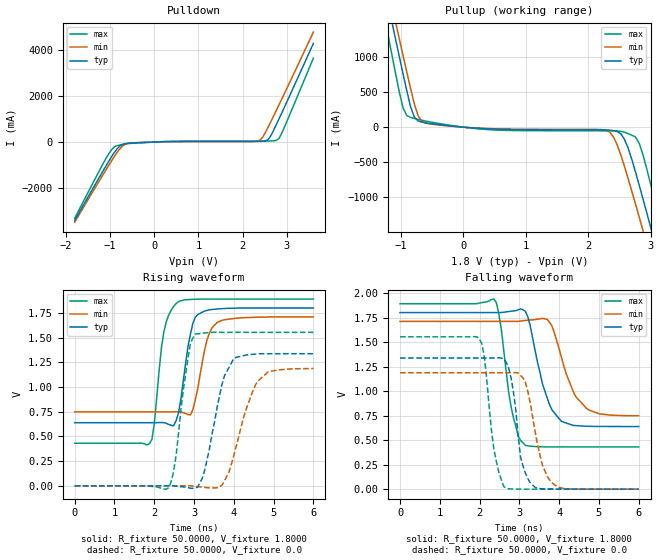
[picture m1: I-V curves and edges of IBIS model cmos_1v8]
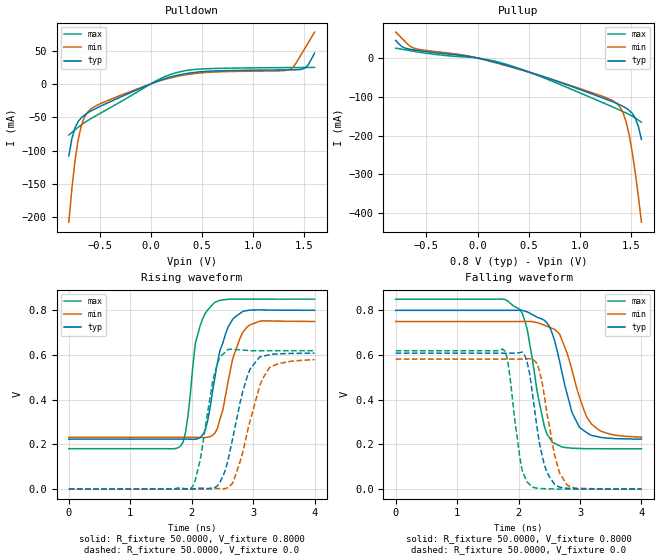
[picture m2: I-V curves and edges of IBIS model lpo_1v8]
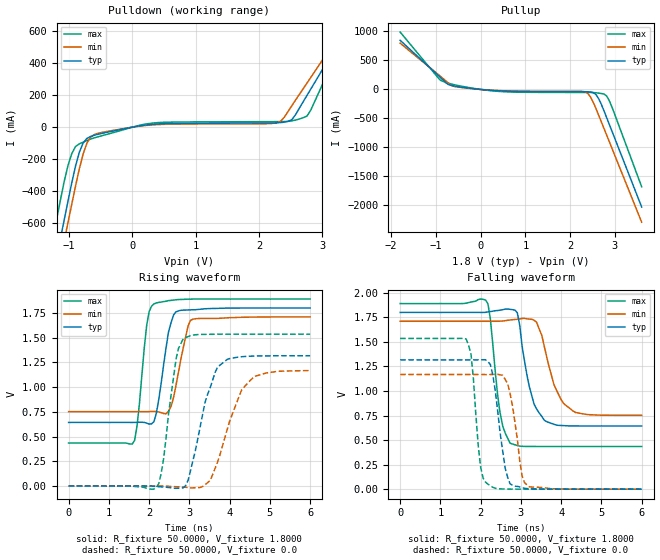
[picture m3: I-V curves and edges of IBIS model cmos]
[IBIS ver]   4.1
[File name]   5l35023.ibs
[File Rev]   1.1
[Date]   Mar 30, 2017
[Source]   IDT
[Notes]   1. Temp typ=25C, max=105C, min=-40C
[Disclaimer]
READ THESE TERMS AND CONDITIONS CAREFULLY BEFORE USING THIS IBIS MODEL.  BY
USING THIS IBIS MODEL, YOU ARE ACCEPTING AND AGREEING TO THESE TERMS AND
CONDITIONS OF USE.
INTEGRATED DEVICE TECHNOLOGY, INC. ("IDT") HEREBY GRANTS THE USER OF THIS
IBIS MODEL ("USER") A NON-EXCLUSIVE, NONTRANSFERABLE LICENSE TO USE THIS
IBIS MODEL UNDER THE FOLLOWING TERMS: THE USER IS GRANTED THIS LICENSE ONLY
TO USE THE IBIS MODEL FOR DEMONSTRATION PURPOSES ONLY AND IS NOT GRANTED
RIGHTS TO SELL, COPY (EXCEPT AS NEEDED TO RUN THE IBIS MODEL), RENT, LEASE
OR SUB-LICENSE (EXCEPT FOR DEMONSTRATION) THE IBIS MODEL IN WHOLE OR IN
PART, OR IN MODIFIED FORM TO ANYONE. THE USER MAY MODIFY THE IBIS MODEL TO
SUIT ITS SPECIFIC APPLICATIONS, BUT  RIGHTS TO DERIVATIVE WORKS AND SUCH
MODIFICATIONS SHALL BELONG TO IDT.
THIS IBIS MODEL IS PROVIDED ON AN AS IS" BASIS AND IDT  MAKES ABSOLUTELY NO
WARRANTY WITH RESPECT TO THE INFORMATION CONTAINED HEREIN.  IDT DISCLAIMS
AND USER WAIVES ALL WARRANTIES, EXPRESS AND IMPLIED, INCLUDING WARRANTIES OF
MERCHANTABILITY AND FITNESS FOR A PARTICULAR PURPOSE.  THE ENTIRE RISK AS TO
QUALITY AND PERFORMANCE IS WITH THE USER  ACCORDINGLY, IN NO EVENT SHALL IDT
BE LIABLE FOR ANY DIRECT OR INDIRECT DAMAGES, WHETHER IN CONTRACT OR TORT,
INCLUDING ANY LOST PROFITS OR OTHER INCIDENTAL, CONSEQUENTIAL, EXEMPLARY, OR
PUNITIVE DAMAGES ARISING OUT OF THE USE OR APPLICATION OF THE  IBIS MODEL,
WHETHER OR NOT IDT HAD NOTICE OF SUCH DAMAGES.
IDT RESERVES THE RIGHT TO MAKE CHANGES WITHOUT NOTICE TO ANY PRODUCT HEREIN
TO IMPROVE RELIABILITY, FUNCTION, OR DESIGN. IDT DOES NOT CONVEY ANY LICENSE
UNDER PATENT RIGHTS OR ANY OTHER INTELLECTUAL PROPERTY RIGHTS, INCLUDING
THOSE OF THIRD PARTIES. IDT IS NOT OBLIGATED TO PROVIDE  MAINTENANCE OR
SUPPORT FOR THE LICENSED IBIS MODEL.
This model is for VC3S 1.8V in 24 pin package
[Copyright]
Copyright 2017, Integrated Device Technology, Inc. All rights  reserved.
|History
|Rev 1.0 Created on Feb 22, 2017
|Rev 1.1 Fixed pinout, Mar 30, 2017
|   Component IDT_vc3s_1p8v
[Component]   IDT_vc3s_1p8v
[Manufacturer]   Integrated Device Technology Inc.
[Package]
| Following package parameters are for the 24 pin QFN package
| variable   typ   min   max
R_pkg   72.4655m   58.886m   86.045m
L_pkg   1.47175nH   1.11650nH   1.77850nH
C_pkg   0.07747pF   0.07444pF   0.08050pF
[Pin]  signal_name   model_name
1   VDDA   POWER
2   SDA   input
3   SCL   input
4   X2   NC
5   XIN   xin
6   VBAT   POWER
7   NC   NC
8   REF   cmos
9   VDD18   POWER
10   OE2   input
11   VDDSE2   POWER
12   SE2   cmos
13   VDDSE1   POWER
14   SE1   cmos
15   OE1   input
16   VDDDIFF1   POWER
17   DIFF1B   IO
18   DIFF1   IO
19   SE3   cmos
20   VDDSE3   POWER
21   OE3   input
22   VDDDIFF2   POWER
23   DIFF2B   IO
24   DIFF2   IO
25   EPAD   GND
[Diff Pin]  inv_pin  vdiff   tdelay_typ  tdelay_min  tdelay_max
18   17   0.000V   0.000s   0.000s   0.000s
24   23   0.000V   0.000s   0.000s   0.000s
[Model Selector] IO
cmos_1v8  1.8V LVCMOS
lpo_1v8   1.8V LP-HCSL
| Models and submodels in the file (5): cmos_1v8 (Output), lpo_1v8 (Output), cmos (Output), input (Input), xin (Input)
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|   Model CMOS_1V8
[Model]  cmos_1v8
Model_type Output
Polarity   Non-Inverting
Vmeas =  0.9000V
Cref =   5.0000pF
Rref =   50.0000
Vref =   0.9000V
C_comp   2.0000pF   1.5000pF   2.5000pF
[Temperature Range]   55.0000   0.1050k   -40.0000
[Voltage Range]   1.8000V   1.7100V   1.8900V
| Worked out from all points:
|   slope of the pulldown table from 0 to 0.27 V, typ, clamps not added: 17.2 ohm
|   slope of the pullup table from 0 to 0.27 V, typ, clamps not added: 15 ohm
|   rising waveform, R_fixture 50.0000, V_fixture 1.8000: 20-80 % time 261ps typ, 293ps min, 242ps max; typ from 0.639 V to 1.8 V
|   rising waveform, R_fixture 50.0000, V_fixture 0.0: 20-80 % time 405ps typ, 518ps min, 280ps max; typ from 0 V to 1.34 V
|   falling waveform, R_fixture 50.0000, V_fixture 1.8000: 20-80 % time 429ps typ, 489ps min, 299ps max; typ from 1.8 V to 0.639 V
|   falling waveform, R_fixture 50.0000, V_fixture 0.0: 20-80 % time 252ps typ, 350ps min, 260ps max; typ from 1.34 V to 0 V
[Pulldown]
|Voltage   I(typ)   I(min)   I(max)
-1.8V     -3.421A    -3.497A    -3.324A
-1.02V    -808.5mA   -987.3mA   -484.5mA
-900mV    -444.5mA   -622.2mA   -206mA
-720mV    -106.4mA   -182.2mA   -104.7mA
-480mV    -39.39mA   -33.93mA   -53.82mA
2.22V     26.08mA    23.46mA    34.43mA
2.4V      30.69mA    93.67mA    34.93mA
2.58V     118.4mA    663.2mA    42.95mA
2.76V     754.3mA    1.372A     69.48mA
2.82V     1A         1.613A     152.6mA
3V        1.752A     2.341A     897.6mA
3.6V      4.301A     4.795A     3.66A
[Pullup]
|Voltage   I(typ)   I(min)   I(max)
-1.8V     4.309A     4.435A     4.081A
-1.26V    2.009A     2.225A     1.584A
-1.14V    1.504A     1.738A     1.036A
-960mV    756.6mA    1.017A     272.1mA
-840mV    290.4mA    550.5mA    138.4mA
-600mV    61.99mA    56.74mA    86.82mA
2.34V     -41.79mA   -66.94mA   -53.12mA
2.58V     -171.4mA   -554.9mA   -72.12mA
2.76V     -645mA     -1.102A    -142.5mA
3V        -1.424A    -1.863A    -812.5mA
3.18V     -2.025A    -2.443A    -1.467A
3.6V      -3.449A    -3.813A    -3.029A
[Ramp]
| variable   typ   min   max
dV/dt_r  0.8022/0.3951n   0.7122/0.5183n   0.9318/0.2801n
dV/dt_f  0.6968/0.4192n   0.5770/0.4887n   0.8755/0.2991n
R_load = 50.0000
[Rising Waveform]
R_fixture= 50.0000
V_fixture= 1.8000
V_fixture_min= 1.7100
V_fixture_max= 1.8900
|time   V(typ)   V(min)   V(max)
0s        638.7mV    748mV      430.9mV
1.88ns    638.6mV    748mV      428.2mV
2ns       638.6mV    748mV      625.1mV
2.24ns    638.9mV    747.9mV    1.555V
2.61ns    741.6mV    749.6mV    1.864V
2.85ns    1.415V     721.5mV    1.884V
3.09ns    1.731V     978.4mV    1.889V
3.33ns    1.775V     1.482V     1.89V
3.58ns    1.79V      1.652V     1.89V
6ns       1.8V       1.71V      1.89V
[Rising Waveform]
R_fixture= 50.0000
V_fixture= 0.0
V_fixture_min= 0.0
V_fixture_max= 0.0
|time   V(typ)   V(min)   V(max)
0s        1.911nV    29.08nV    578.9pV
2.36ns    1.233mV    -18.22uV   -18.94mV
2.55ns    -4.157mV   -34.61uV   309.9mV
2.91ns    -24.11mV   84.21uV    1.442V
3.03ns    -20.99mV   -7.045mV   1.536V
3.27ns    161.3mV    -15.27mV   1.547V
3.7ns     1.018V     4.261mV    1.553V
4ns       1.289V     309.7mV    1.554V
4.61ns    1.336V     1.061V     1.553V
6ns       1.337V     1.187V     1.553V
[Falling Waveform]
R_fixture= 50.0000
V_fixture= 1.8000
V_fixture_min= 1.7100
V_fixture_max= 1.8900
|time   V(typ)   V(min)   V(max)
0s        1.8V       1.71V      1.89V
2.36ns    1.8V       1.71V      1.938V
2.55ns    1.801V     1.71V      1.621V
2.79ns    1.814V     1.71V      842.9mV
3.15ns    1.814V     1.72V      448mV
3.7ns     930.9mV    1.731V     430.6mV
4.06ns    690.5mV    1.341V     431.1mV
4.36ns    649.9mV    990mV      430.7mV
4.73ns    640.9mV    810.5mV    430.9mV
6ns       638.7mV    748.4mV    430.9mV
[Falling Waveform]
R_fixture= 50.0000
V_fixture= 0.0
V_fixture_min= 0.0
V_fixture_max= 0.0
|time   V(typ)   V(min)   V(max)
0s        1.337V     1.187V     1.553V
2ns       1.337V     1.187V     1.526V
2.12ns    1.336V     1.187V     1.345V
2.36ns    1.337V     1.187V     409.2mV
2.67ns    1.294V     1.187V     9.479mV
3.03ns    326.3mV    1.159V     248.5uV
3.33ns    42.9mV     748.3mV    1.743uV
3.58ns    3.646mV    244.4mV    611.1nV
3.88ns    779.1uV    45.72mV    -433nV
6ns       909.2nV    -18.83uV   442.8nV
|   Model LPO_1V8
[Model]  lpo_1v8
Model_type Output
Polarity   Non-Inverting
Vmeas =  0.4000V
Cref =   2.0000pF
Rref =   0.0
Vref =   0.4000V
C_comp   2.0000pF   1.5000pF   2.5000pF
[Temperature Range]   55.0000   0.1050k   -40.0000
[Voltage Range]   0.8000V   0.7500V   0.8500V
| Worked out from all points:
|   slope of the pulldown table from 0 to 0.12 V, typ, clamps not added: 17.3 ohm
|   slope of the pullup table from 0 to 0.12 V, typ, clamps not added: 16.3 ohm
|   rising waveform, R_fixture 50.0000, V_fixture 0.8000: 20-80 % time 258ps typ, 264ps min, 191ps max; typ from 0.223 V to 0.8 V
|   rising waveform, R_fixture 50.0000, V_fixture 0.0: 20-80 % time 301ps typ, 330ps min, 221ps max; typ from 0 V to 0.608 V
|   falling waveform, R_fixture 50.0000, V_fixture 0.8000: 20-80 % time 315ps typ, 354ps min, 253ps max; typ from 0.8 V to 0.224 V
|   falling waveform, R_fixture 50.0000, V_fixture 0.0: 20-80 % time 212ps typ, 232ps min, 169ps max; typ from 0.608 V to 0 V
[Pulldown]
|Voltage   I(typ)   I(min)   I(max)
-800mV    -108.1mA   -207.2mA   -76.54mA
-770mV    -81.98mA   -157mA     -72.66mA
-740mV    -65.89mA   -115.8mA   -68.83mA
-710mV    -56.66mA   -84.79mA   -65.13mA
-650mV    -47.11mA   -50.8mA    -58.4mA
-590mV    -41.16mA   -38.34mA   -52.61mA
40mV      2.523mA    2.167mA    3.578mA
250mV     12.51mA    10.98mA    16.76mA
580mV     19.07mA    17.47mA    22.88mA
1.36V     21mA       21.81mA    24.43mA
1.51V     24.16mA    54.42mA    24.58mA
1.6V      46.14mA    77.6mA     24.67mA
[Pullup]
|Voltage   I(typ)   I(min)   I(max)
-800mV    45.53mA    67mA       25.2mA
-740mV    29.62mA    51.3mA     22.99mA
-620mV    20.88mA    25.41mA    17.24mA
-110mV    5.14mA     6.271mA    2.571mA
220mV     -14.15mA   -15.38mA   -11.61mA
1.06V     -87.09mA   -84.22mA   -96.78mA
1.36V     -117.3mA   -117.6mA   -131mA
1.42V     -124.8mA   -141.1mA   -138.1mA
1.48V     -134.9mA   -198.4mA   -145.7mA
1.54V     -155.3mA   -297mA     -155mA
1.57V     -176.6mA   -357.7mA   -160.3mA
1.6V      -210mA     -423.7mA   -165.9mA
[Ramp]
| variable   typ   min   max
dV/dt_r  0.3649/0.3012n   0.3475/0.3303n   0.3716/0.2211n
dV/dt_f  0.3457/0.3147n   0.3101/0.3539n   0.4016/0.2533n
R_load = 50.0000
[Rising Waveform]
R_fixture= 50.0000
V_fixture= 0.8000
V_fixture_min= 0.7500
V_fixture_max= 0.8500
|time   V(typ)   V(min)   V(max)
0s        223.4mV    231.5mV    180.7mV
1.82ns    223.5mV    231.5mV    192.8mV
1.9ns     223.5mV    231.5mV    254.5mV
2.06ns    223mV      231.4mV    653.1mV
2.1ns     225.2mV    231.2mV    693mV
2.26ns    305.9mV    232mV      801.5mV
2.42ns    567.6mV    272.3mV    840.5mV
2.67ns    761.6mV    585.9mV    850.4mV
2.95ns    801.2mV    735mV      850.2mV
4ns       800.1mV    750.3mV    850mV
[Rising Waveform]
R_fixture= 50.0000
V_fixture= 0.0
V_fixture_min= 0.0
V_fixture_max= 0.0
|time   V(typ)   V(min)   V(max)
0s        2.542nV    41nV       676.4pV
1.98ns    -230.8uV   22.6uV     1.542mV
2.14ns    3.82mV     -261uV     132.6mV
2.38ns    7.63mV     3.333mV    525.4mV
2.59ns    127.8mV    6.862mV    624.7mV
2.67ns    230.3mV    27.37mV    625.5mV
2.83ns    436.7mV    162.3mV    622.2mV
3.07ns    579.2mV    424.5mV    619mV
3.27ns    601.4mV    544.2mV    619.2mV
4ns       608.2mV    579.1mV    619.3mV
[Falling Waveform]
R_fixture= 50.0000
V_fixture= 0.8000
V_fixture_min= 0.7500
V_fixture_max= 0.8500
|time   V(typ)   V(min)   V(max)
0s        800mV      750mV      850mV
2.02ns    800.3mV    750mV      804.5mV
2.14ns    793mV      750.3mV    716.7mV
2.38ns    761.3mV    737.9mV    332.4mV
2.51ns    724.3mV    723.7mV    227.7mV
2.67ns    568.9mV    692.4mV    193.7mV
2.87ns    342.9mV    531.3mV    183.3mV
2.99ns    277.3mV    412.4mV    182mV
3.31ns    233.5mV    263.9mV    180.9mV
4ns       223.9mV    233.1mV    180.7mV
[Falling Waveform]
R_fixture= 50.0000
V_fixture= 0.0
V_fixture_min= 0.0
V_fixture_max= 0.0
|time   V(typ)   V(min)   V(max)
0s        608.5mV    581.8mV    619.3mV
1.78ns    608.5mV    581.8mV    616.8mV
2.06ns    613.1mV    581.7mV    81.97mV
2.14ns    568.5mV    583.1mV    32.35mV
2.22ns    439.6mV    583.8mV    9.709mV
2.34ns    205.4mV    528.8mV    3.658mV
2.46ns    76.86mV    341.5mV    1.545mV
2.63ns    13.87mV    109.2mV    565.6uV
2.79ns    4.079mV    17.95mV    165.5uV
4ns       15.08uV    69.86uV    273.2nV
|   Model CMOS
[Model]  cmos
Model_type Output
Polarity   Non-Inverting
Vmeas =  0.9000V
Cref =   5.0000pF
Rref =   50.0000
Vref =   0.9000V
C_comp   2.0000pF   1.5000pF   2.5000pF
[Temperature Range]   55.0000   0.1050k   -40.0000
[Voltage Range]   1.8000V   1.7100V   1.8900V
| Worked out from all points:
|   slope of the pulldown table from 0 to 0.27 V, typ, clamps not added: 17.3 ohm
|   slope of the pullup table from 0 to 0.27 V, typ, clamps not added: 15.8 ohm
|   rising waveform, R_fixture 50.0000, V_fixture 1.8000: 20-80 % time 251ps typ, 282ps min, 202ps max; typ from 0.643 V to 1.8 V
|   rising waveform, R_fixture 50.0000, V_fixture 0.0: 20-80 % time 472ps typ, 570ps min, 281ps max; typ from 0 V to 1.32 V
|   falling waveform, R_fixture 50.0000, V_fixture 1.8000: 20-80 % time 324ps typ, 415ps min, 235ps max; typ from 1.8 V to 0.643 V
|   falling waveform, R_fixture 50.0000, V_fixture 0.0: 20-80 % time 248ps typ, 242ps min, 182ps max; typ from 1.32 V to 0 V
[Pulldown]
|Voltage   I(typ)   I(min)   I(max)
-1.8V     -1.999A    -2.094A    -1.823A
-1.26V    -936.5mA   -1.059A    -704.5mA
-1.08V    -582.3mA   -713.4mA   -341.8mA
-1.02V    -464.5mA   -598.3mA   -241.7mA
-840mV    -157.5mA   -261.4mA   -104.6mA
-660mV    -58.08mA   -61.8mA    -74.43mA
360mV     18.73mA    15.09mA    26.94mA
2.28V     26.73mA    26.9mA     34.29mA
2.52V     46.83mA    133.9mA    39.32mA
2.76V     198.6mA    275.4mA    69.19mA
3.42V     638.5mA    668.1mA    631.7mA
3.6V      760.8mA    777.4mA    791.6mA
[Pullup]
|Voltage   I(typ)   I(min)   I(max)
-1.8V     847.6mA    798.1mA    988.7mA
-960mV    249.7mA    265.7mA    208.6mA
-780mV    116.5mA    147.4mA    122.3mA
-600mV    60.31mA    53.77mA    83.72mA
-120mV    9.611mA    7.962mA    14.15mA
660mV     -31.39mA   -25.96mA   -44mA
2.22V     -38.37mA   -32.38mA   -51.99mA
2.4V      -40.59mA   -72.13mA   -52.3mA
2.58V     -89.45mA   -332.8mA   -57.45mA
2.82V     -491.7mA   -792.7mA   -115.8mA
2.94V     -727.8mA   -1.023A    -312.5mA
3.6V      -2.027A    -2.288A    -1.678A
[Ramp]
| variable   typ   min   max
dV/dt_r  0.7902/0.4623n   0.7002/0.5702n   0.9210/0.2714n
dV/dt_f  0.6941/0.3351n   0.5747/0.4153n   0.8732/0.2314n
R_load = 50.0000
[Rising Waveform]
R_fixture= 50.0000
V_fixture= 1.8000
V_fixture_min= 1.7100
V_fixture_max= 1.8900
|time   V(typ)   V(min)   V(max)
0s        643.2mV    752.1mV    434.6mV
1.64ns    643.4mV    752.1mV    461.8mV
1.76ns    645.2mV    752mV      834.8mV
1.94ns    635.8mV    752.3mV    1.625V
2.12ns    650.7mV    754.1mV    1.841V
2.24ns    876.3mV    749.2mV    1.856V
2.48ns    1.553V     755.4mV    1.874V
2.67ns    1.761V     1.023V     1.883V
3.03ns    1.781V     1.675V     1.889V
6ns       1.8V       1.71V      1.89V
[Rising Waveform]
R_fixture= 50.0000
V_fixture= 0.0
V_fixture_min= 0.0
V_fixture_max= 0.0
|time   V(typ)   V(min)   V(max)
0s        1.498nV    35.29nV    34.1pV
2.18ns    -5.295mV   205.9uV    -11.27mV
2.36ns    -9.254mV   823.4uV    274.8mV
2.67ns    -22.86mV   -6.794mV   1.285V
2.85ns    -17.53mV   -10.54mV   1.49V
3.33ns    725.4mV    -4.525mV   1.533V
3.7ns     1.202V     241.9mV    1.535V
4.3ns     1.307V     972.8mV    1.535V
4.61ns    1.314V     1.107V     1.535V
6ns       1.317V     1.167V     1.535V
[Falling Waveform]
R_fixture= 50.0000
V_fixture= 1.8000
V_fixture_min= 1.7100
V_fixture_max= 1.8900
|time   V(typ)   V(min)   V(max)
0s        1.8V       1.71V      1.89V
2.12ns    1.801V     1.71V      1.927V
2.24ns    1.809V     1.71V      1.737V
2.48ns    1.823V     1.711V     782mV
2.73ns    1.832V     1.723V     468mV
2.91ns    1.797V     1.73V      444.4mV
3.21ns    1.042V     1.732V     434.8mV
3.58ns    702.3mV    1.456V     434.6mV
4.3ns     644mV      794.6mV    434.6mV
6ns       643.2mV    752.1mV    434.6mV
[Falling Waveform]
R_fixture= 50.0000
V_fixture= 0.0
V_fixture_min= 0.0
V_fixture_max= 0.0
|time   V(typ)   V(min)   V(max)
0s        1.317V     1.168V     1.535V
1.64ns    1.317V     1.168V     1.529V
1.76ns    1.317V     1.168V     1.375V
2ns       1.318V     1.168V     222.6mV
2.3ns     1.165V     1.168V     19.46mV
2.61ns    211.9mV    1.117V     1.137mV
2.73ns    55.42mV    975.7mV    309.2uV
3.03ns    15.79mV    132.2mV    -29.19uV
3.21ns    4.108mV    23.6mV     -358.7nV
6ns       -48.98uV   26.04uV    274.1nV
